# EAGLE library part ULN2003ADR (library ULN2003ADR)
Trans Darlington NPN 50V 0.5A SOIC16 Texas Instruments ULN2003ADR, 7-element NPN Darlington Transistor Array, 0.5 A 50 V, 16-Pin SOIC Source: Datasheet
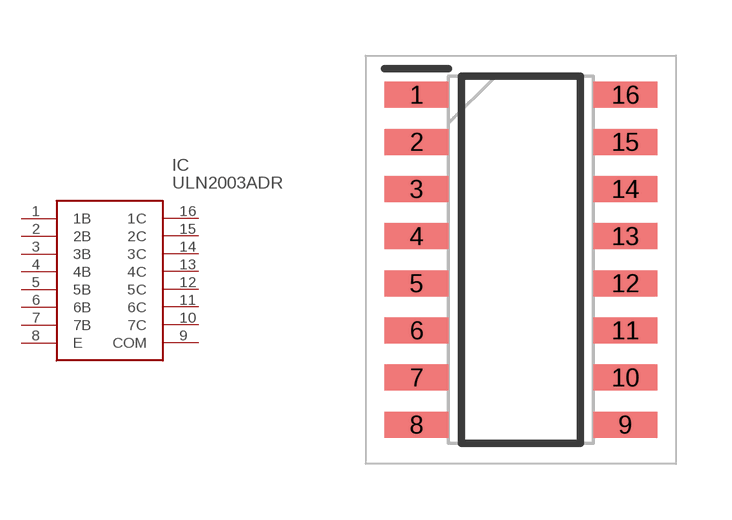
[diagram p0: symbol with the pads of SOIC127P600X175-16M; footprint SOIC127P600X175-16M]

Designator prefix IC

## ULN2003ADR (Description: Trans Darlington NPN 50V 0.5A SOIC16 Texas Instruments ULN2003ADR, 7-element NPN Darlington Transistor Array, 0.5 A 50 V, 16-Pin SOIC; Height: 1.75mm; Manufacturer_Name: Texas Instruments; Manufacturer_Part_Number: ULN2003ADR; Mouser_Part_Number: 595-ULN2003ADR; Mouser_Price-Stock: https://www.mouser.co.uk/ProductDetail/Texas-Instruments/ULN2003ADR?qs=D5pVkbrsqqI8WxXD0eSvDA%3D%3D)  [SOIC127P600X175-16M]
1  1B
2  2B
3  3B
4  4B
5  5B
6  6B
7  7B
8  E
9  COM
10  7C
11  6C
12  5C
13  4C
14  3C
15  2C
16  1C

## Footprint SOIC127P600X175-16M (pad centres in mm)
D (R-PDSO-G16)
smd 1.725 x 0.7: 1 -2.812,4.445; 2 -2.812,3.175; 3 -2.812,1.905; 4 -2.812,0.635; 5 -2.812,-0.635; 6 -2.812,-1.905; 7 -2.812,-3.175; 8 -2.812,-4.445; 9 2.812,-4.445; 10 2.812,-3.175; 11 2.812,-1.905; 12 2.812,-0.635; 13 2.812,0.635; 14 2.812,1.905; 15 2.812,3.175; 16 2.812,4.445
